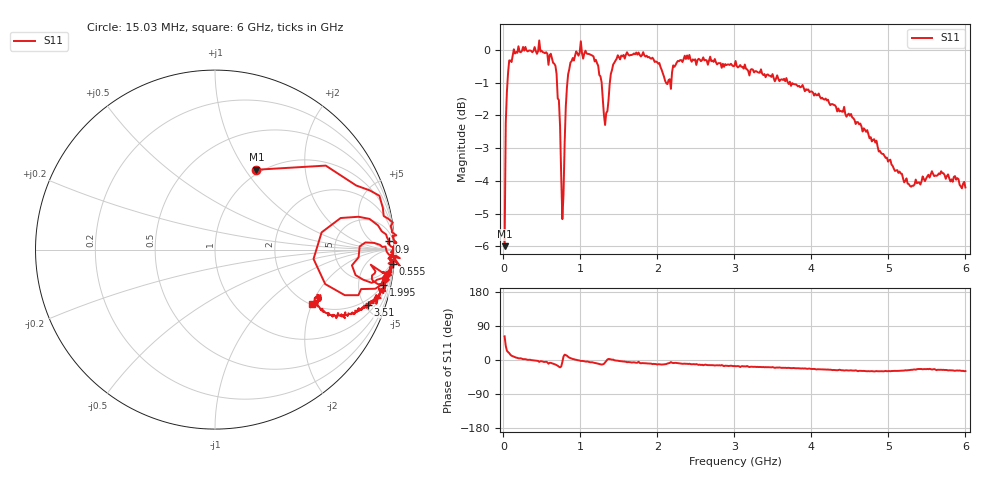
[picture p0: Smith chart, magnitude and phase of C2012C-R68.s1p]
!	Network	Analyzer	HP8753E.07.74:	Oct	30	2002	Serial	No.	JP38451487
!	Hewlett-Packard
!	28	Aug	2009	12:47:42
!	Frequency	S11
#	HZ	S	RI	R	50
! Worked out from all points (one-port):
!   400 points, 15.03 MHz to 6 GHz, reference 50 ohm
!   lowest |S11| = -6.0 dB at 15.03 MHz (marker M1), VSWR 3.01, Z = 47.4 + j56.4 ohm
!   |S11| at or under -10 dB: nowhere
!   S11 on the Smith chart (normalised r, x): 15.03 MHz: 0.95, +1.13; 555 MHz: 3, -25; 900 MHz: 19, +31; 1.995 GHz: 1.91, -9.24; 3.51 GHz: 1.55, -5.29; 6 GHz: 2.04, -1.98
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1.502992e7  0.231 0.445
3.002985e7  0.617 0.468
4.502978e7  0.787 0.357
7.502962e7  0.916 0.3
1.95029e8  1.01 0.0795
5.550272e8  0.989 -0.0781
6.750266e8  0.925 -0.197
7.350263e8  0.723 -0.254
7.650262e8  0.549 -0.0521
7.95026e8  0.7 0.176
8.400258e8  0.908 0.135
9.000255e8  0.971 0.0457
1.005025e9  1.03 -0.0478
1.200024e9  0.956 -0.138
1.275024e9  0.873 -0.185
1.320023e9  0.763 -0.088
1.365023e9  0.838 0.0399
1.425023e9  0.95 0.0171
1.515022e9  0.966 -0.0497
1.99502e9  0.938 -0.197
2.175019e9  0.868 -0.0843
2.265019e9  0.952 -0.139
3.015015e9  0.923 -0.271
3.510012e9  0.852 -0.307
3.765011e9  0.828 -0.319
4.515007e9  0.71 -0.365
5.265004e9  0.557 -0.281
6e9  0.538 -0.301
